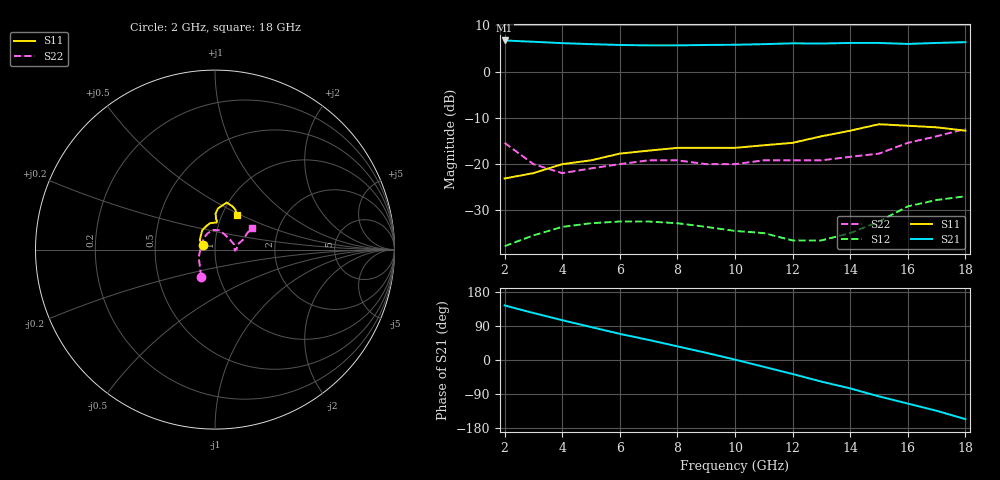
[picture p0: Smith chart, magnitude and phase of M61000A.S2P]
!  MGA-61000 S PARAMETERS
!  Vd=5V, Id=80mA  LAST UPDATED 07-22-92
# ghz s ma r 50
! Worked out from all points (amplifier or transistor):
!   17 points, 2 GHz to 18 GHz, reference 50 ohm
!   highest |S21| = 6.7 dB at 2 GHz (marker M1)
!   |S21| within 3 dB of that: start of sweep to end of sweep
!   unconditionally stable (mu >= 1): start of sweep to end of sweep
!   at 4 GHz: K = 11.57, MAG = 6.2 dB, |S12| = -33.6 dB
!   at 10 GHz: K = 13.09, MAG = 5.9 dB, |S12| = -34.4 dB
!   at 18 GHz: K = 4.76, MAG = 6.9 dB, |S12| = -26.9 dB
2  0.07 158.0  2.17 144.0  0.013 56.0  0.17 -117.0
3  0.08 158.0  2.1 124.0  0.017 51.0  0.1 -155.0
4  0.1 148.0  2.03 105.0  0.021 46.0  0.08 164.0
5  0.11 136.0  1.98 87.0  0.023 39.0  0.09 133.0
6  0.13 123.0  1.94 69.0  0.024 30.0  0.1 114.0
7  0.14 110.0  1.92 53.0  0.024 22.0  0.11 95.0
8  0.15 101.0  1.92 36.0  0.023 13.0  0.11 78.0
9  0.15 91.0  1.94 19.0  0.021 6.0  0.1 57.0
10  0.15 87.0  1.95 1.0  0.019 -5.0  0.1 34.0
11  0.16 86.0  1.98 -18.0  0.018 -14.0  0.11 15.0
12  0.17 88.0  2.02 -37.0  0.015 -14.0  0.11 2.0
13  0.2 89.0  2.01 -57.0  0.015 -28.0  0.11 -3.0
14  0.23 86.0  2.04 -75.0  0.018 -35.0  0.12 1.0
15  0.27 76.0  2.04 -96.0  0.024 -45.0  0.13 13.0
16  0.26 68.0  1.99 -115.0  0.035 -68.0  0.17 20.0
17  0.25 63.0  2.04 -134.0  0.041 -89.0  0.2 27.0
18  0.23 58.0  2.08 -156.0  0.045 -111.0  0.24 30.0
